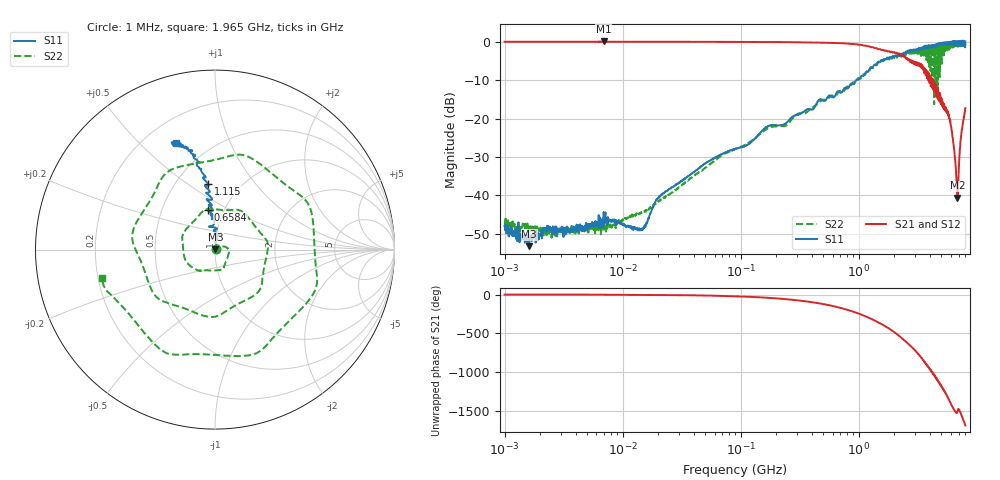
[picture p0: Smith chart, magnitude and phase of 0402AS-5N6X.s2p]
!s-Parameter Generated by FASTRON Sdn. Bhd.
!FASTRON P/N : 0402AS-5N6X
!Keysight Technologies: E5071C_MY46733604_B.14.02
!Date: Mon Dec 01 10:24:48 2025
!Version  :Rev00  Mon Dec 01 10:24:48 2025
!Data & Calibration Information:
!Freq  S11:SOLT2(ON)  S21:SOLT2(ON)  S12:SOLT2(ON)  S22:SOLT2(ON)
!PortZ  Port1:50+j0  Port2:50+j0
!When reading reference impedance value at option line is always used.
! Remarks : This data is being provided solely for informational purposes.
# Hz S dB R 50
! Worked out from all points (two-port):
!   1601 points, 1 MHz to 8 GHz, reference 50 ohm
!   highest |S21| = 0.04 dB at 6.912 MHz (marker M1); lowest = -40.6 dB at 6.843 GHz (marker M2)
!   |S21| within 3 dB of the highest: start of sweep to 2.028 GHz; 2.074 GHz to 2.109 GHz (35.73 MHz wide, 1.71 % of centre)
!   lowest |S11| = -53.2 dB at 1.614 MHz (marker M3), VSWR 1.00, Z = 50.2 + j0.0918 ohm
!   |S11| at or under -10 dB: start of sweep to 951.7 MHz
!   |S22| runs from -51.2 to -0.4 dB; largest |S21 - S12| = 0.017
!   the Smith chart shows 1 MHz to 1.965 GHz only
!   S11 on the Smith chart (normalised r, x): 1 MHz: 1.01, +0.00; 658.4 MHz: 0.84, +0.39; 1.115 GHz: 0.71, +0.61; 1.965 GHz: 0.33, +0.65
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1000000  -47.90 20.3  -0.05 -0.3  -0.02 -0.3  -46.80 16.1
1613744  -53.20 24.7  -0.04 -0.4  -0.03 -0.4  -48.00 -0.3
4479405  -47.90 29.9  -0.05 -1.1  -0.03 -1.2  -48.60 35.9
6911657  -44.30 9.6  0.04 -2.2  0.03 -2.0  -45.60 18.2
2.00676e7  -40.70 43.9  -0.05 -5.1  -0.04 -5.0  -41.50 64.5
8.994653e7  -27.90 89.3  -0.08 -22.5  -0.07 -22.4  -28.00 27.8
4.006501e8  -17.70 101.0  -0.22 -98.9  -0.21 -98.9  -17.30 -123.0
6.583697e8  -13.00 100.0  -0.39 -162.0  -0.39 -162.0  -13.60 116.0
1.114569e9  -8.64 96.1  -0.99 84.9  -0.98 84.8  -8.66 -107.0
1.45009e9  -5.31 103.0  -1.93 3.2  -1.92 3.1  -5.53 80.7
1.7949e9  -4.41 108.0  -2.46 -77.3  -2.46 -77.4  -4.52 -84.1
1.96534e9  -3.98 110.0  -2.87 -118.0  -2.88 -118.0  -3.75 -166.0
2.178389e9  -3.77 114.0  -3.07 -169.0  -3.07 -169.0  -3.82 88.3
2.354847e9  -3.29 118.0  -3.69 148.0  -3.67 148.0  -3.04 0.2
2.560258e9  -2.92 120.0  -4.32 99.3  -4.30 99.2  -2.79 -101.0
2.89772e9  -2.10 128.0  -5.51 18.5  -5.49 18.4  -2.72 82.8
3.26428e9  -2.16 136.0  -5.60 -68.4  -5.57 -68.7  -3.52 -92.8
3.60885e9  -1.56 145.0  -7.85 -147.0  -7.82 -147.0  -1.08 97.0
3.973689e9  -1.01 149.0  -10.80 121.0  -10.80 121.0  -4.09 -112.0
4.324643e9  -1.49 155.0  -10.70 35.9  -10.70 35.4  -3.64 132.0
6.843354e9  -0.11 -110.0  -40.60 -71.4  -40.60 -71.6  -0.94 0.1
8e9  0.01 -91.6  -17.30 109.0  -17.40 109.0  -1.31 151.0
